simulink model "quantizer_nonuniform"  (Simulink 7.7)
settings: Solver=FixedStepDiscrete  StartTime=0.0  StopTime=10  FixedStep=1/fs  RelTol=1e-3
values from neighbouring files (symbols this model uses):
  A = 87.6    [quantizer_test.m]
  k = sqrt(10^(atenuation/10))    [quantizer_test.m]
undefined symbols (not defined in the file or in its folder): fs
libraries: commsrccod2 x2, dspquant2 x1, dspsrcs4 x1

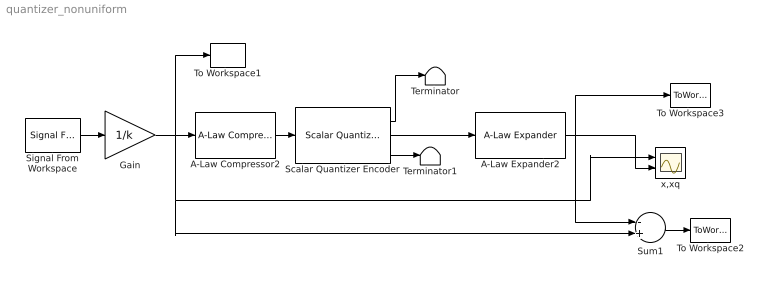
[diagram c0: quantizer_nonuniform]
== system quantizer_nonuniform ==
  A-Law Compressor2 : commsrccod2/A-Law Compressor  SystemSampleTime=-1  A=A  V=1
  A-Law Expander2 : commsrccod2/A-Law Expander  SystemSampleTime=-1  A=A  V=1
  Gain : Gain  Gain=1/k
  Scalar Quantizer Encoder : dspquant2/Scalar Quantizer Encoder  paramSrc=Specify via dialog  partType=Bounded  BBoundary=boundary  UBoundary=[2:9]  SearchMethod=Linear  tieBreakRule=Choose the lower index  outQU=on  outQError=on  codebook=codebook  outStatus=off  invalidin=Clip  idtype=int32  roundingMode=Floor  overflowMode=off
  Signal From Workspace : dspsrcs4/Signal From Workspace  SystemSampleTime=-1  X=x  Ts=1/fs  nsamps=1  OutputAfterFinalValue=Setting to zero  ignoreOrWarnInputAndFrameLengths=off
  Sum1 : Sum  Inputs=-+
  Terminator : Terminator
  Terminator1 : Terminator
  To Workspace1 : ToWorkspace  VariableName=xout  SampleTime=-1  SaveFormat=Array
  To Workspace2 : ToWorkspace  VariableName=eq  SampleTime=-1  SaveFormat=Array
  To Workspace3 : ToWorkspace  VariableName=xq  SampleTime=-1  SaveFormat=Array
  x,xq : Scope  NumInputPorts=2
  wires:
  Signal From Workspace/1 -> Gain/1
  Scalar Quantizer Encoder/2 -> A-Law Expander2/1
  Scalar Quantizer Encoder/1 -> Terminator/1
  Scalar Quantizer Encoder/3 -> Terminator1/1
  Gain/1 -> To Workspace1/1, Sum1/2, x,xq/1, A-Law Compressor2/1
  Sum1/1 -> To Workspace2/1
  A-Law Compressor2/1 -> Scalar Quantizer Encoder/1
  A-Law Expander2/1 -> Sum1/1, To Workspace3/1, x,xq/2
